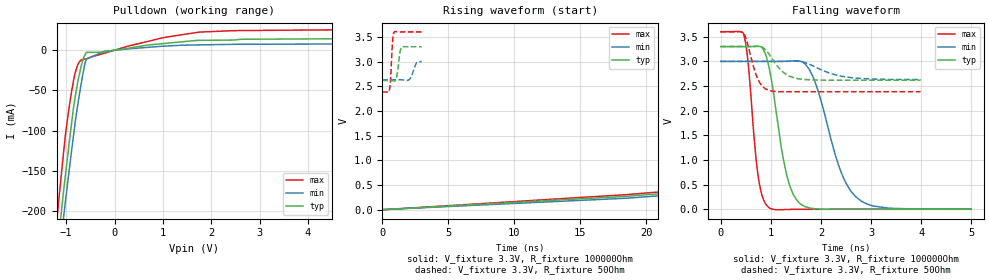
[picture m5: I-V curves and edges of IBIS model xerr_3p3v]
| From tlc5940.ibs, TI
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|   xerr_3p3v Model
[Model]   xerr_3p3v
Model_type   Open_drain
Polarity   Inverting
Vmeas = 1.65
Vref = 3.3
Cref = 15pF
Rref = 100000
|   typ   min   max
|   (nom PVT)   (Fast PVT)   (slow PVT)
|Average
C_comp   1.172e-12   1.163e-12   1.175e-12
|ON state : BUFFER OUTPUT TURNED LOW
|C_comp   1.280e-12   1.276e-12   1.295e-12
|OFF state: BUFFER in HIGH IMPEDANCE
|C_comp   1.056e-12   1.051e-12   1.063e-12
| Where nom  PVT is Nominal Process, 3.3V, 65C
|   Fast PVT is Strong Process,  3.6V, -40C
|   Slow PVT is Weak Process,   3V, 125C
[Voltage Range]   3.3   3   3.6
|Ambient Temperature   25   85   -40
|Junction Temperature
[Temperature Range]   65   125   -40
[Pullup Reference]   3.3   3   3.6
[Pulldown Reference]   0   0   0
[Power Clamp Reference]   3.3   3   3.6
[GND Clamp Reference]   0   0   0
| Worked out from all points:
|   slope of the pulldown table from 0 to 0.495 V, typ, clamps not added: 110 ohm
|   falling waveform, V_fixture 3.3V, R_fixture 100000Ohm: 20-80 % time 316ps typ, 523ps min, 186ps max; typ from 3.3 V to 0.004 V
|   rising waveform, V_fixture 3.3V, R_fixture 100000Ohm: 20-80 % time 155ns typ, 153ns min, 155ns max; typ from 0.003 V to 3.3 V
|   rising waveform, V_fixture 3.3V, R_fixture 50Ohm: 20-80 % time 191ps typ, 292ps min, 142ps max; typ from 2.62 V to 3.3 V
|   falling waveform, V_fixture 3.3V, R_fixture 50Ohm: 20-80 % time 330ps typ, 578ps min, 211ps max; typ from 3.3 V to 2.62 V
[Pulldown]
|   Voltage   I(typ)   I(min)   I(max)
-3.3V     -1.556A    -1.491A    -1.677A
-1.191V   -251.9mA   -279.9mA   -210.9mA
-1.167V   -238.4mA   -266.9mA   -195.5mA
-1.147V   -227.4mA   -256.6mA   -182.9mA
-1.043V   -169.4mA   -202.2mA   -120.7mA
-949.2mV  -121mA     -155.1mA   -75mA
-823.2mV  -61.7mA    -94.27mA   -30.24mA
-693mV    -20.61mA   -42.68mA   -12.4mA
-584.1mV  -2.741mA   -11.11mA   -10.57mA
-213mV    -2.463mA   -1.36mA    -3.777mA
1.751V    12.26mA    6.612mA    22.53mA
6.6V      14.94mA    8.177mA    26.32mA
[Ramp]
R_load = 100000
|   typ   min   max
dV/dt_r   1.97811/1.54933e-07   1.79708/1.52996e-07   2.15884/1.55275e-07
dV/dt_f   1.97769/3.16406e-10   1.7963/5.21693e-10   2.15843/1.85879e-10
[Falling Waveform]
V_fixture = 3.3V
V_fixture_min = 3V
V_fixture_max = 3.6V
R_fixture = 100000Ohm
|   Time   V(typ)   V(min)   V(max)
0s        3.3V       3V         3.6V
460ps     3.3V       3V         3.537V
750ps     3.306V     3V         657.3mV
970ps     2.852V     2.999V     31.1mV
1.31ns    726.4mV    3.002V     -2.13mV
1.6ns     105.2mV    3V         2.596mV
1.84ns    18.5mV     2.689V     2.755mV
2.35ns    4.355mV    901.2mV    2.695mV
2.69ns    4.191mV    261.2mV    2.683mV
5ns       3.821mV    6.088mV    2.611mV
[Rising Waveform]
V_fixture = 3.3V
V_fixture_min = 3V
V_fixture_max = 3.6V
R_fixture = 100000Ohm
|   Time   V(typ)   V(min)   V(max)
0s        3.099mV    4.764mV    1.894mV
18.52ns   274.5mV    235.6mV    308.6mV
47.17ns   841.5mV    781.2mV    913.4mV
80.58ns   1.42V      1.317V     1.547V
133.7ns   2.134V     1.957V     2.325V
199ns     2.681V     2.45V      2.921V
276.4ns   3.017V     2.749V     3.289V
363.1ns   3.185V     2.898V     3.473V
489.5ns   3.27V      2.973V     3.566V
1us       3.3V       3V         3.6V
[Rising Waveform]
V_fixture = 3.3V
V_fixture_min = 3V
V_fixture_max = 3.6V
R_fixture = 50Ohm
|   Time   V(typ)   V(min)   V(max)
0s        2.618V     2.631V     2.385V
540ps     2.619V     2.631V     2.424V
620ps     2.619V     2.631V     2.638V
780ps     2.614V     2.631V     3.43V
910ps     2.606V     2.631V     3.602V
1.08ns    2.686V     2.632V     3.603V
1.43ns    3.281V     2.631V     3.599V
2.07ns    3.3V       2.644V     3.599V
2.59ns    3.3V       2.974V     3.599V
2.99ns    3.3V       2.999V     3.6V
[Falling Waveform]
V_fixture = 3.3V
V_fixture_min = 3V
V_fixture_max = 3.6V
R_fixture = 50Ohm
|   Time   V(typ)   V(min)   V(max)
0s        3.3V       3V         3.6V
450ps     3.3V       3V         3.583V
520ps     3.3V       3V         3.413V
740ps     3.305V     3V         2.645V
830ps     3.286V     3V         2.499V
970ps     3.138V     3V         2.41V
1.25ns    2.779V     3.001V     2.385V
1.55ns    2.648V     3.001V     2.385V
2.5ns     2.618V     2.684V     2.385V
3.99ns    2.618V     2.632V     2.385V
